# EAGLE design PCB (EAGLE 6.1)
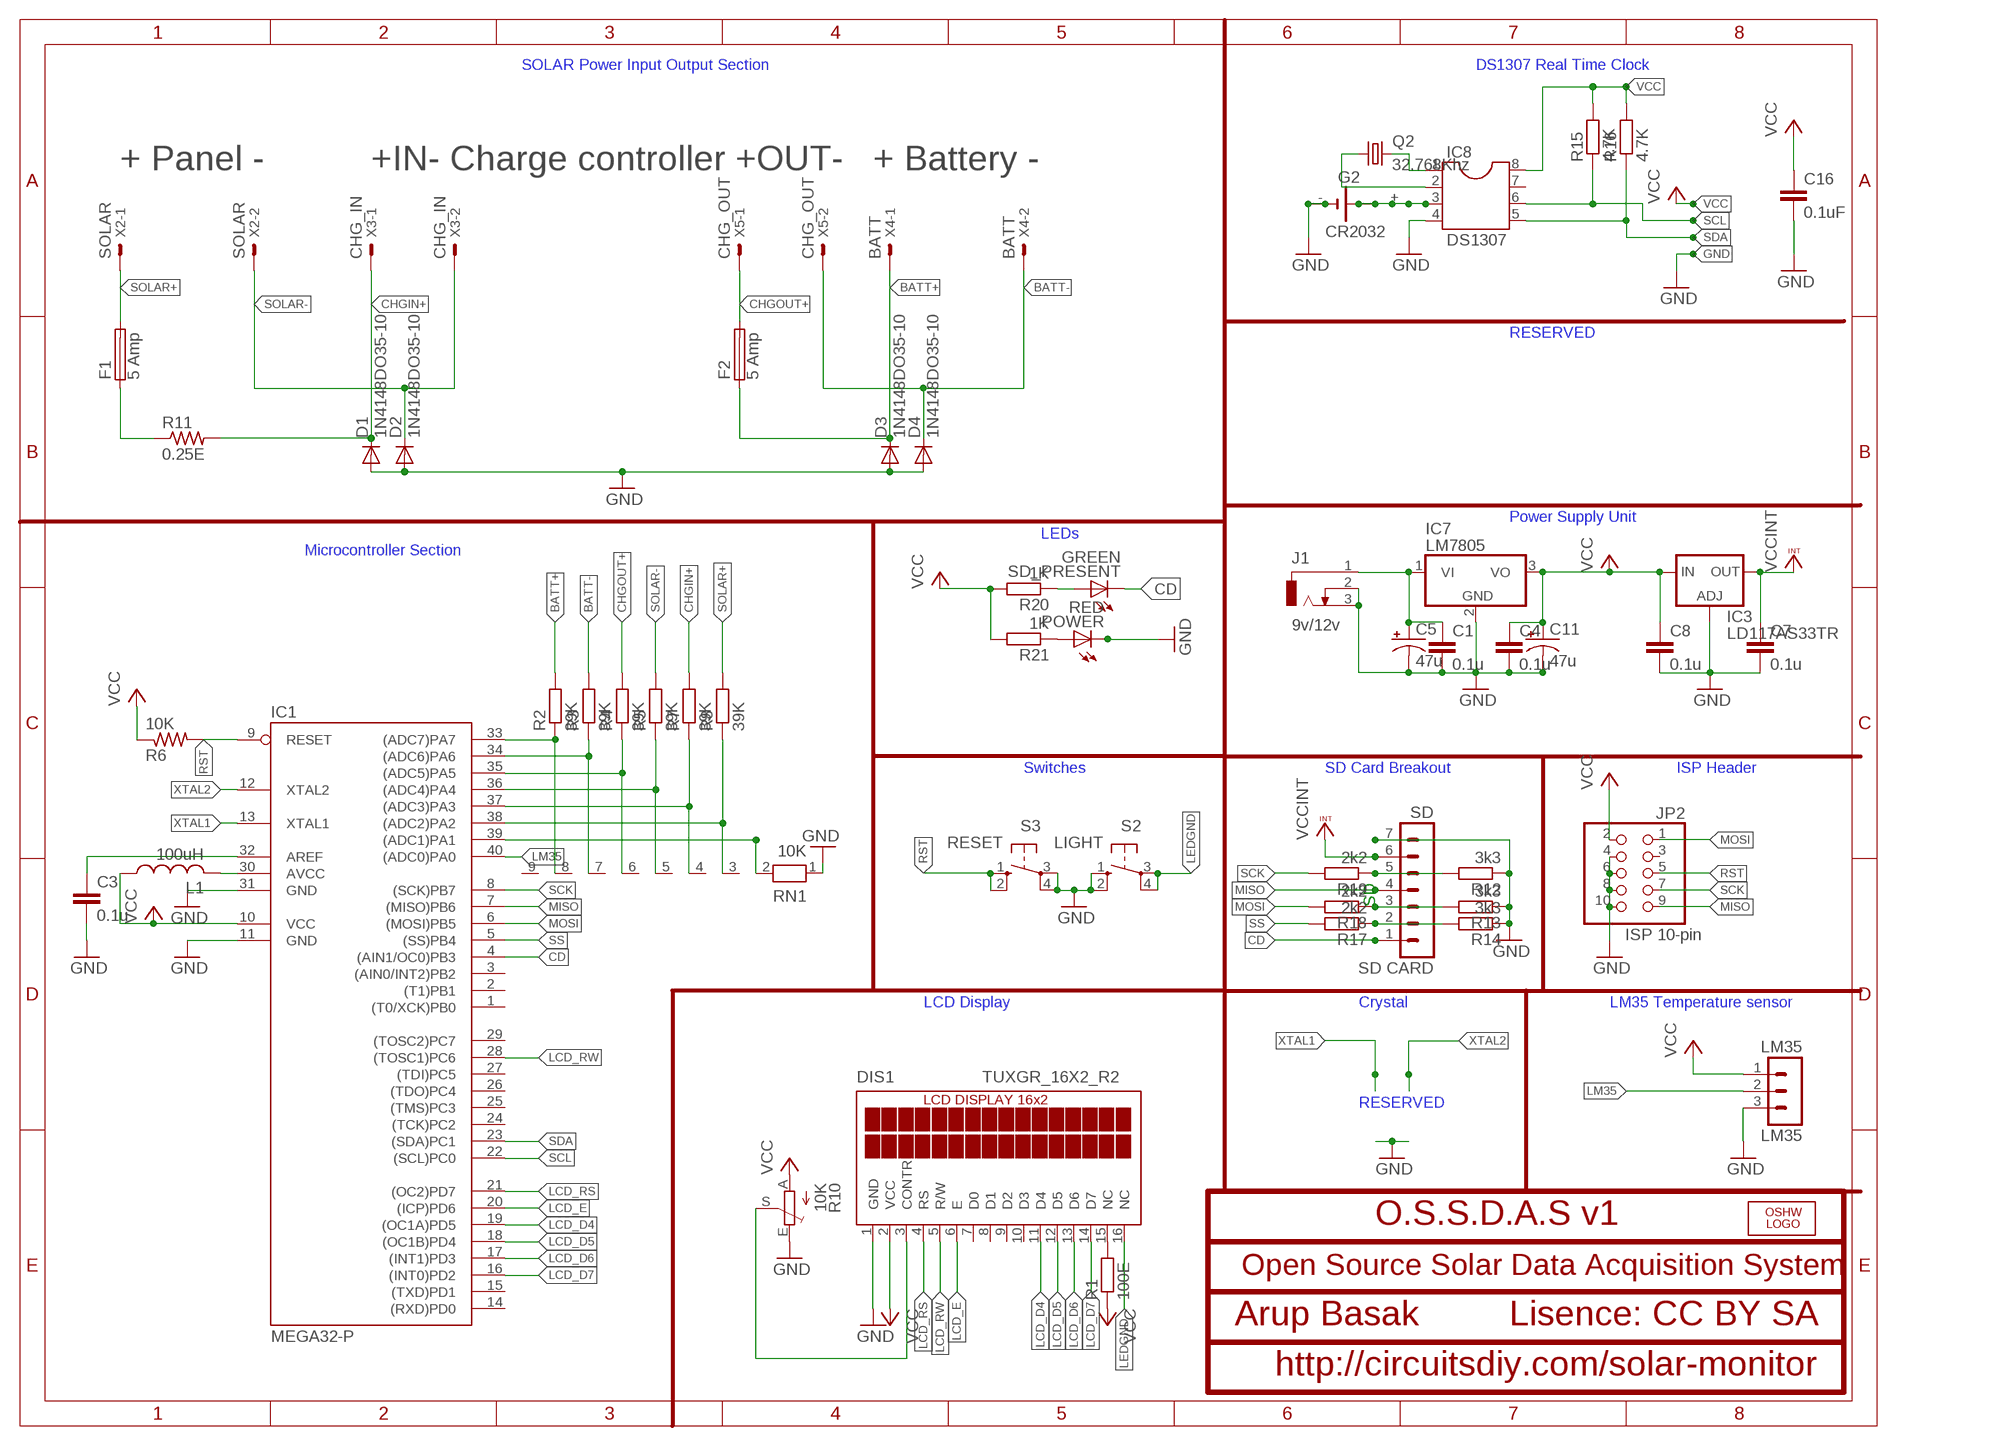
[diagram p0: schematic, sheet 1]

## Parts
C1  0.1u  C-EU025-025X050  [C025-025X050]
C3  0.1u  C-EU025-025X050  [C025-025X050]
C4  0.1u  C-EU025-025X050  [C025-025X050]
C5  47u  CPOL-USE2.5-7  [E2,5-7]
C7  0.1u  C-EU025-025X050  [C025-025X050]
C8  0.1u  C-EU025-025X050  [C025-025X050]
C11  47u  CPOL-USE2.5-7  [E2,5-7]
C16  0.1uF  C-EU050-024X044  [C050-024X044]
D1  1N4148DO35-10  [DO35-10]
D2  1N4148DO35-10  [DO35-10]
D3  1N4148DO35-10  [DO35-10]
D4  1N4148DO35-10  [DO35-10]
DIS1  TUXGR_16X2_R2  [TUXGR_16X2_R2]
F1  5 Amp  SH22,5A  [SH22,5A]
F2  5 Amp  SH22,5A  [SH22,5A]
G2  CR2032  B2430UNI  [B2430UNI]
IC1  MEGA32-P  [DIL40]
IC3  LD117AS33TR  [SOT223]
IC7  LM7805  7805TV  [TO220V]
IC8  DS1307  DIL8  [DIL08]
J1  9v/12v  DCJ0202  [DCJ0202]
JP2  ISP 10-pin  PINHD-2X5  [2X05]
L1  100uH  L-US0207/12  [0207/12]
LM35  LM35  MA03-1  [MA03-1]
LOGO1  OSHW_LOGO_FILLX0350-NT  [OSHW_FILLX350_NOTEXT]
POWER  RED  LED5MM  [LED5MM]
Q2  32.768Khz  CRYSTALTC38H  [TC38H]
R1  100E  R-EU_0207/7  [0207/7]
R2  39K  R-EU_0207/10  [0207/10]
R3  39K  R-EU_0207/10  [0207/10]
R4  39K  R-EU_0207/10  [0207/10]
R5  39K  R-EU_0207/10  [0207/10]
R6  10K  R-US_0207/10  [0207/10]
R7  39K  R-EU_0207/10  [0207/10]
R8  39K  R-EU_0207/10  [0207/10]
R10  10K  TRIM_EU-CA6V  [CA6V]
R11  0.25E  R-US_VTA53  [VTA53]
R12  3k3  R-EU_0207/10  [0207/10]
R13  3k3  R-EU_0207/10  [0207/10]
R14  3k3  R-EU_0207/10  [0207/10]
R15  4.7K  R-EU_0207/7  [0207/7]
R16  4.7K  R-EU_0207/7  [0207/7]
R17  2k2  R-EU_0207/10  [0207/10]
R18  2k2  R-EU_0207/10  [0207/10]
R19  2k2  R-EU_0207/10  [0207/10]
R20  1K  R-EU_0207/10  [0207/10]
R21  1K  R-EU_0207/10  [0207/10]
RN1  10K  RN08  [RN-9]
S2  LIGHT  10-XX  [B3F-10XX]
S3  RESET  10-XX  [B3F-10XX]
SD  SD CARD  MA07-1  [MA07-1]
SD_PRESENT  GREEN  LED5MM  [LED5MM]
X2  SOLAR  KK-156-2  [KK-156-2]
X3  CHG_IN  KK-156-2  [KK-156-2]
X4  BATT  KK-156-2  [KK-156-2]
X5  CHG_OUT  KK-156-2  [KK-156-2]

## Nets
AREF: C3.1 IC1.32(AREF)
AVCC: IC1.30(AVCC) L1.2
BATT+: D3.C F2.1 R2.2 X4.1
BATT-: D4.C R3.2 X4.2 X5.2
CD: IC1.4((AIN1/OC0)PB3) SD.1 SD_PRESENT.K(C)
CHGIN+: D1.C R7.2 R11.2 X3.1
CHGOUT+: F2.2 R4.2 X5.1
CS: R14.2 R17.1 SD.2
D1: R13.2 R18.1 SD.3
GND: C1.2 C3.2 C4.2 C5.- C7.2 C8.2 C11.- C16.2 D1.A D2.A D3.A D4.A DIS1.1(GND) G2.- G2.-@1(-) IC1.11(GND) IC1.31(GND) IC3.1(ADJ) IC7.2(GND) IC8.4 J1.2 J1.3 JP2.4 JP2.6 JP2.8 JP2.10 LM35.3 POWER.K(C) R10.E R12.1 R13.1 R14.1 RN1.1 S2.1(S) S2.2(S1) S3.3(P) S3.4(P1) SD.7
LCD_D4: DIS1.11(D4) IC1.19((OC1A)PD5)
LCD_D5: DIS1.12(D5) IC1.18((OC1B)PD4)
LCD_D6: DIS1.13(D6) IC1.17((INT1)PD3)
LCD_D7: DIS1.14(D7) IC1.16((INT0)PD2)
LCD_E: DIS1.6(E) IC1.20((ICP)PD6)
LCD_RS: DIS1.4(RS) IC1.21((OC2)PD7)
LCD_RW: DIS1.5(R/W) IC1.28((TOSC1)PC6)
LEDGND: DIS1.16(NC) S2.3(P) S2.4(P1)
LM35: IC1.40((ADC0)PA0) LM35.2
MISO: IC1.7((MISO)PB6) JP2.9 SD.4
MOSI: IC1.6((MOSI)PB5) JP2.1 R18.2
N$2: DIS1.15(NC) R1.2
N$3: IC1.33((ADC7)PA7) R2.1 RN1.8
N$4: DIS1.3(CONTR) R10.S
N$5: IC1.34((ADC6)PA6) R3.1 RN1.7
N$6: IC1.35((ADC5)PA5) R4.1 RN1.6
N$7: IC1.36((ADC4)PA4) R5.1 RN1.5
N$8: IC8.1 Q2.2
N$9: IC1.37((ADC3)PA3) R7.1 RN1.4
N$10: IC1.38((ADC2)PA2) R8.1 RN1.3
N$11: IC1.39((ADC1)PA1) RN1.2
N$12: IC8.2 Q2.1
N$16: G2.+ G2.+@1(+) G2.+@2(+) G2.+@3(+) G2.+@4(+) IC8.3
N$17: F1.1 R11.1
N$22: R20.1 SD_PRESENT.A
N$23: POWER.A R21.1
N$24: C1.1 C5.+ IC7.1(VI) J1.1
RST: IC1.9(RESET) JP2.5 R6.2 S3.1(S) S3.2(S1)
SCK: IC1.8((SCK)PB7) JP2.7 R19.2
SCL: IC1.22((SCL)PC0) IC8.6 R15.1
SD_SCK: R12.2 R19.1 SD.5
SDA: IC1.23((SDA)PC1) IC8.5 R16.1
SOLAR+: F1.2 R8.2 X2.1
SOLAR-: D2.C R5.2 X2.2 X3.2
SS: IC1.5((SS)PB4) R17.2
VCC: C4.1 C8.1 C11.+ C16.1 DIS1.2(VCC) IC1.10(VCC) IC3.3(IN) IC7.3(VO) IC8.8 JP2.2 L1.1 LM35.1 R1.1 R6.1 R10.A R15.2 R16.2 R20.2 R21.2
VCCINT: C7.1 IC3.4(OUT) SD.6
XTAL1: IC1.13(XTAL1)
XTAL2: IC1.12(XTAL2)
Unconnected: DIS1.7(D0) DIS1.8(D1) DIS1.9(D2) DIS1.10(D3) IC1.1((T0/XCK)PB0) IC1.2((T1)PB1) IC1.3((AIN0/INT2)PB2) IC1.14((RXD)PD0) IC1.15((TXD)PD1) IC1.24((TCK)PC2) IC1.25((TMS)PC3) IC1.26((TDO)PC4) IC1.27((TDI)PC5) IC1.29((TOSC2)PC7) IC8.7 JP2.3 RN1.9

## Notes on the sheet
- SOLAR Power Input Output Section | DS1307 Real Time Clock
- + Panel - | +IN- Charge controller +OUT- | + Battery -
- RESERVED
- Power Supply Unit
- LEDs
- Microcontroller Section
- Switches | SD Card Breakout | ISP Header
- SD
- LCD Display | Crystal | LM35 Temperature sensor
- RESERVED
- O.S.S.D.A.S v1
- Open Source Solar Data Acquisition System
- Arup Basak | Lisence: CC BY SA
- http://circuitsdiy.com/solar-monitor

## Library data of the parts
C1 C3 C4 C7 C8 = resistor:C-EU: CAPACITOR, European symbol
C5 C11 = resistor:CPOL-US: POLARIZED CAPACITOR, American symbol
C16 = rcl:C-EU: CAPACITOR, European symbol
D1-D4 = diode:1N4148: DIODE
DIS1 = display-lcd:TUXGR_16X2_R2: Tuxgraphics LCD display 16x2 characters reflective, without background light Source: tuxgr_12x2_r2.pdf; OC_FARNELL: unknown; OC_NEWARK: unknown
F1 F2 = fuse:SH22,5A: FUSE HOLDER; MPN: 0031.7701.11; OC_FARNELL: unknown; OC_NEWARK: 04F1224
G2 = battery:B2430UNI: LI BATTERY
IC1 = atmel:MEGA32-P: MICROCONTROLLER 32 Kbytes FLASH 2 Kbytes SRAM 1 Kbytes EEPROM USART 8-channel 10 bit ADC Source: www.atmel.com .. doc2503.pdf
IC3 = v-reg:LD117A?*: Low drop fixed and adjustable positive voltage regulators 1 A Source: http://www.st.com/stonline/products/literature/ds/7194/ld1117axx.pdf
IC7 = linear:78*: Positive VOLTAGE REGULATOR Source: http://cache.national.com/ds/LM/LM78L05.pdf http://www.fairchildsemi.com/ds/LM/LM7805.pdf
IC8 = ic-package:DIL8: Dual In Line / Socket
J1 = con-jack:DCJ0202: DC POWER JACK Source: DCJ0202.pdf
JP2 = sonar:PINHD-2X5: PIN HEADER
L1 = resistor:L-US: INDUCTOR, American symbol
LM35 = con-lstb:MA03-1: PIN HEADER
LOGO1 = ohw-logo:OSHW_LOGO_FILL
POWER SD_PRESENT = led:LED: LED
Q2 = crystal:CRYSTAL: CRYSTAL
R1-R5 R7 R8 R15 R16 R20 R21 = rcl:R-EU_: RESISTOR, European symbol
R6 = resistor:R-US_: RESISTOR, American symbol
R10 = pot:TRIM_EU-: POTENTIOMETER
R11 = rcl:R-US_: RESISTOR, American symbol
R12-R14 R17-R19 = resistor:R-EU_: RESISTOR, European symbol
RN1 = resistor-net:RN08: RESISTOR NETWORK
S2 S3 = switch-omron:10-XX: OMRON SWITCH
SD = con-lstb:MA07-1: PIN HEADER
X2-X5 = con-molex:KK-156-2: KK 156 HEADER; OC_FARNELL: unknown; OC_NEWARK: unknown

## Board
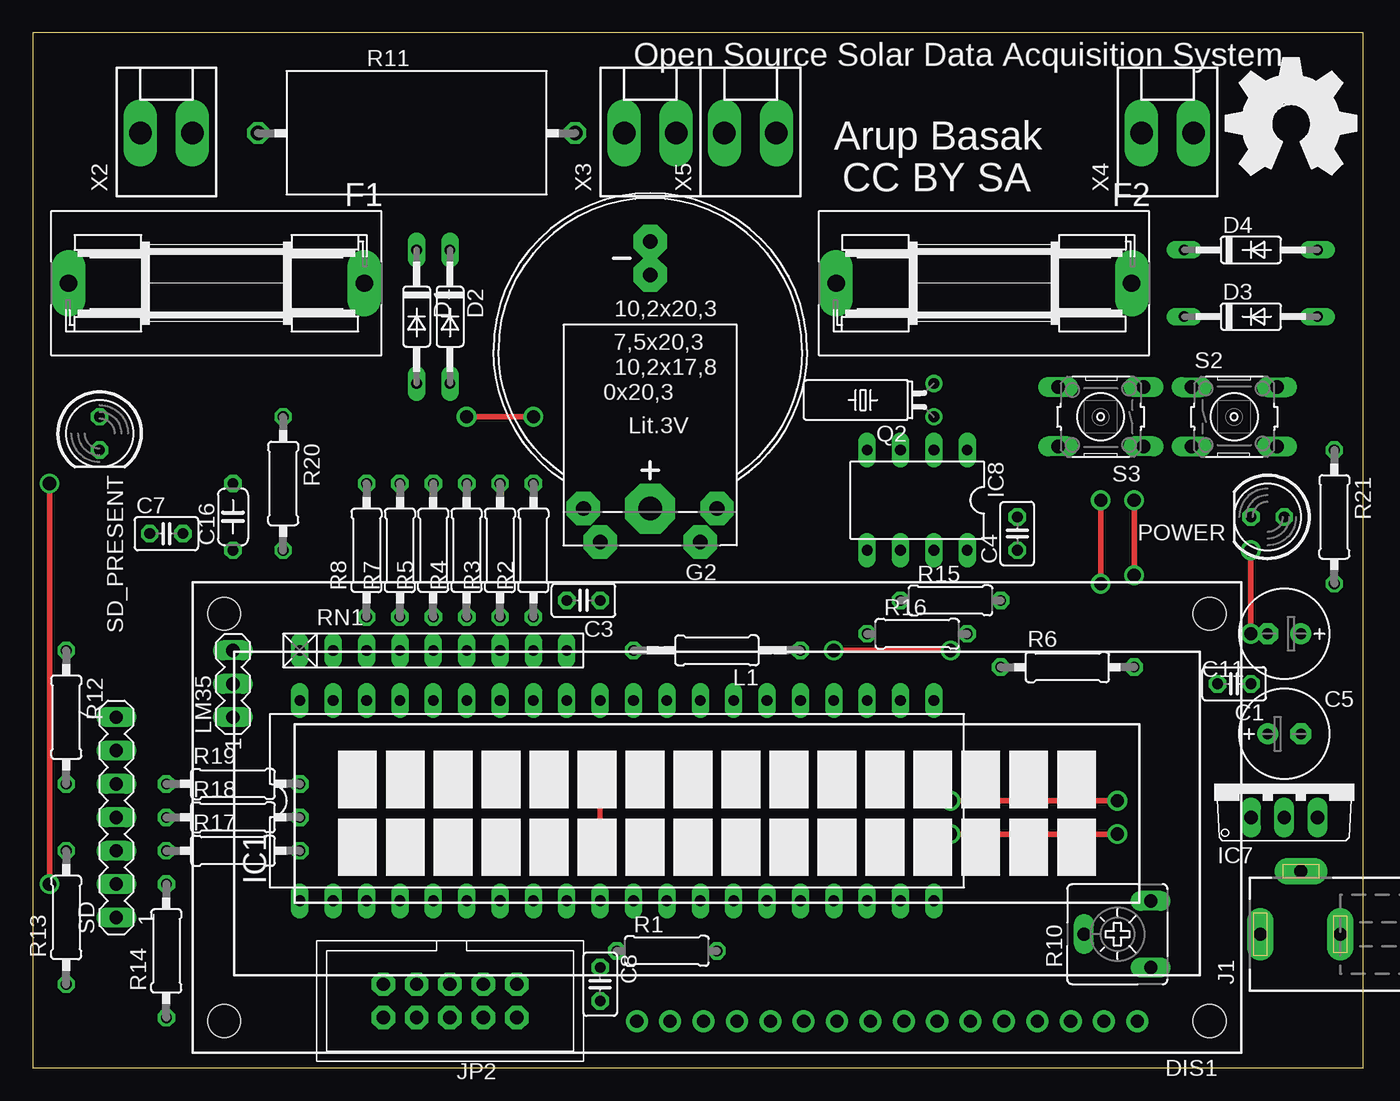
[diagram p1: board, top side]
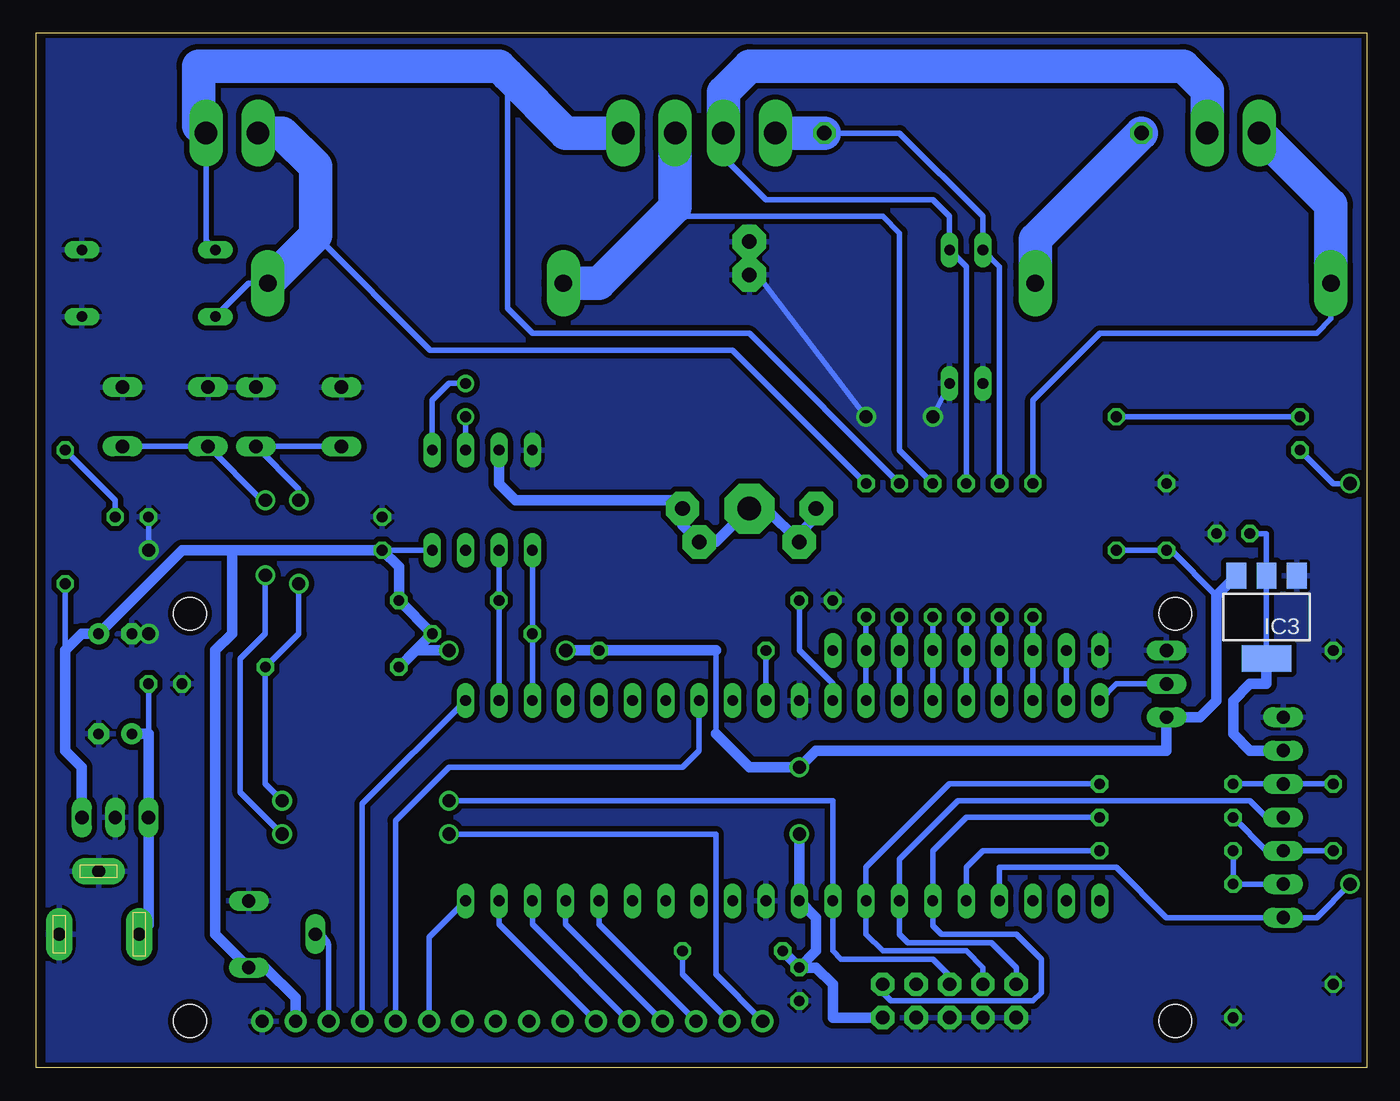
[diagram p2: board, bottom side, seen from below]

Size 101.27 x 78.73 mm. Coordinates in mm from the lower left corner, seen from the top.
Outline: 0,0 101.27,0 101.27,78.73 0,78.73 0,0
Copper layers (1*16): Top 0.035mm / dielectric 1.5mm / Bottom 0.035mm
Design rules: minimum track width 6mil, minimum drill 12mil, track to track 6mil, track to pad 6mil, pad to pad 6mil, via to via 6mil, smd to smd 0mil, copper to edge 10mil, drill to drill 10mil, minimum pad ring 10mil, minimum via ring 6mil, stop-mask expansion 2mil, vias tented up to drill 100mil, thermal gap 10mil

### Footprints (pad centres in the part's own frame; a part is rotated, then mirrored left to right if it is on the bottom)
C025-025X050 = drill 0.813 octagon: 1 -1.27,0; 2 1.27,0
E2,5-7 = drill 0.813 pad 1.6: + -1.27,0 | drill 0.813 pad 1.6 octagon: - 1.27,0
C050-024X044 = drill 0.813 octagon: 1 -2.54,0; 2 2.54,0
DO35-10 = drill 0.813 long: A 5.08,0; C -5.08,0
TUXGR_16X2_R2 = drill 1 pad 1.676: 1 -32,15.5; 2 -29.46,15.5; 3 -26.92,15.5; 4 -24.38,15.5; 5 -21.84,15.5; 6 -19.3,15.5; 7 -16.76,15.5; 8 -14.22,15.5; 9 -11.68,15.5; 10 -9.14,15.5; 11 -6.6,15.5; 12 -4.06,15.5; 13 -1.52,15.5; 14 1.02,15.5; 15 3.56,15.5; 16 6.1,15.5 | hole 2.5: -37.5,-15.5; 37.5,-15.5; -37.5,15.5; 37.5,15.5
SH22,5A = drill 1.321 pad 2.54 long: 1 -11.252,0; 2 11.252,0
B2430UNI = drill 1.118 pad 2.54 octagon: + 3.81,14.605; +@1 -3.81,14.605; +@2 -5.08,12.065; +@3 5.08,12.065; - 0,-5.715; -@1 0,-8.255 | drill 1.803 pad 3.81 octagon: +@4 0,12.065
DIL40 = drill 0.813 long: 1 -24.13,-7.62; 2 -21.59,-7.62; 3 -19.05,-7.62; 4 -16.51,-7.62; 5 -13.97,-7.62; 6 -11.43,-7.62; 7 -8.89,-7.62; 8 -6.35,-7.62; 9 -3.81,-7.62; 10 -1.27,-7.62; 11 1.27,-7.62; 12 3.81,-7.62; 13 6.35,-7.62; 14 8.89,-7.62; 15 11.43,-7.62; 16 13.97,-7.62; 17 16.51,-7.62; 18 19.05,-7.62; 19 21.59,-7.62; 20 24.13,-7.62; 21 24.13,7.62; 22 21.59,7.62; 23 19.05,7.62; 24 16.51,7.62; 25 13.97,7.62; 26 11.43,7.62; 27 8.89,7.62; 28 6.35,7.62; 29 3.81,7.62; 30 1.27,7.62; 31 -1.27,7.62; 32 -3.81,7.62; 33 -6.35,7.62; 34 -8.89,7.62; 35 -11.43,7.62; 36 -13.97,7.62; 37 -16.51,7.62; 38 -19.05,7.62; 39 -21.59,7.62; 40 -24.13,7.62
SOT223 = smd 1.5 x 2: 1 -2.3,-3.15; 2 0,-3.15; 3 2.3,-3.15 | smd 3.8 x 2: 4 0,3.15
TO220V = drill 1.016 long: 1 -2.54,-2.54; 2 0,-2.54; 3 2.54,-2.54
DIL08 = drill 0.813 long: 1 -3.81,-3.81; 2 -1.27,-3.81; 3 1.27,-3.81; 4 3.81,-3.81; 5 3.81,3.81; 6 1.27,3.81; 7 -1.27,3.81; 8 -3.81,3.81
DCJ0202 = drill 1 pad 2 long: 1 0,3.1; 2 4.8,0; 3 0,-3
2X05 = drill 1.016 pad 1.778 octagon: 1 -5.08,-1.27; 2 -5.08,1.27; 3 -2.54,-1.27; 4 -2.54,1.27; 5 0,-1.27; 6 0,1.27; 7 2.54,-1.27; 8 2.54,1.27; 9 5.08,-1.27; 10 5.08,1.27
0207/12 = drill 0.813 octagon: 1 -6.35,0; 2 6.35,0
MA03-1 = drill 1.016 long: 1 -2.54,0; 2 0,0; 3 2.54,0
LED5MM = drill 0.813 octagon: A -1.27,0; K 1.27,0
TC38H = drill 0.813: 1 -1.27,0; 2 1.27,0
0207/7 = drill 0.813 octagon: 1 -3.81,0; 2 3.81,0
0207/10 = drill 0.813 octagon: 1 -5.08,0; 2 5.08,0
CA6V = drill 1.016 long: A -2.54,-2.54; E 2.54,-2.54; S 0,2.54
VTA53 = drill 1.1 octagon: 1 -12.065,0; 2 12.065,0
RN-9 = drill 0.813 long: 1 -10.16,0; 2 -7.62,0; 3 -5.08,0; 4 -2.54,0; 5 0,0; 6 2.54,0; 7 5.08,0; 8 7.62,0; 9 10.16,0
B3F-10XX = drill 1.016 long: 1 -3.251,2.261; 2 3.251,2.261; 3 -3.251,-2.261; 4 3.251,-2.261
MA07-1 = drill 1.016 long: 1 -7.62,0; 2 -5.08,0; 3 -2.54,0; 4 0,0; 5 2.54,0; 6 5.08,0; 7 7.62,0
KK-156-2 = drill 1.7 pad 2.184 long: 1 -1.98,0; 2 1.98,0

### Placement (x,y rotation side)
C1  91.44,29.21 180 top
C3  41.91,35.56 180 top
C4  74.93,40.64 90 top
C5  95.25,25.4 0 top
C7  10.16,40.64 0 top
C8  43.18,6.35 270 top
C11  95.25,33.02 180 top
C16  15.24,41.91 90 top
D1  29.21,57.15 270 top
D2  31.75,57.15 270 top
D3  92.71,57.15 0 top
D4  92.71,62.23 0 top
DIS1  52.07,19.05 180 top
F1  13.97,59.69 180 top
F2  72.39,59.69 180 top
G2  46.99,54.61 180 top
IC1  44.45,20.32 0 top
IC3  7.62,34.29 180 bottom
IC7  95.25,21.59 0 top
IC8  67.31,43.18 180 top
J1  96.52,10.16 90 top
JP2  31.75,5.08 180 top
L1  52.07,31.75 180 top
LM35  15.24,29.21 90 top
LOGO1  90.81,67.95 0 top
POWER  93.98,41.91 180 top
Q2  68.58,50.8 90 top
R1  48.26,8.89 0 top
R2  38.1,39.37 90 top
R3  35.56,39.37 90 top
R4  33.02,39.37 90 top
R5  30.48,39.37 90 top
R6  78.74,30.48 0 top
R7  27.94,39.37 90 top
R8  25.4,39.37 90 top
R10  82.55,10.16 90 top
R11  29.21,71.12 0 top
R12  2.54,26.67 270 top
R13  2.54,11.43 90 top
R14  10.16,8.89 90 top
R15  69.85,35.56 0 top
R16  67.31,33.02 0 top
R17  15.24,16.51 0 top
R18  15.24,19.05 0 top
R19  15.24,21.59 0 top
R20  19.05,44.45 270 top
R21  99.06,41.91 270 top
RN1  30.48,31.75 0 top
S2  91.44,49.53 0 top
S3  81.28,49.53 180 top
SD  6.35,19.05 90 top
SD_PRESENT  5.08,48.26 270 top
X2  10.16,71.12 0 top
X3  46.99,71.12 0 top
X4  86.36,71.12 0 top
X5  54.61,71.12 0 top

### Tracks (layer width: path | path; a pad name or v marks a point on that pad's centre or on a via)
AREF
  Bottom 0.406: IC1.32 40.64,29.21 43.18,31.75 C3.1
AVCC
  Bottom 0.406: L1.2 IC1.30
BATT+
  Bottom 0.406: 80.01,63.32 71.3,54.61 48.26,54.61 R2.2 | 83.64,60.78 F2.1 85.09,59.69 D3.C
  Bottom 2.54: F2.1 80.01,63.32 80.01,68.58 82.55,71.12 X4.1
BATT-
  Bottom 0.406: R3.2 46.99,55.88 63.5,55.88 65.41,57.78 65.41,75.56 | D4.C 88.34,62.94 X4.2
  Bottom 2.54: X5.2 60.96,71.12 65.41,75.56 66.04,76.2 88.9,76.2 88.9,71.68 X4.2
CD  (via drill 1 pad 1.27)
  Top 0.406: v1.27,44.45 v1.27,13.97
  Bottom 0.406: IC1.4 27.94,15.24 19.05,15.24 15.24,11.43 SD.1 3.81,11.43 v1.27,13.97 | SD_PRESENT.K 2.54,44.45 v1.27,44.45
CHGIN+
  Bottom 0.406: R11.2 35.56,71.12 29.21,64.77 D1.C 27.94,60.96 R7.2
  Bottom 2.54: R11.2 X3.1
CHGOUT+
  Bottom 0.406: R4.2 35.56,46.99 35.56,63.5 36.83,64.77 52.07,64.77 52.63,65.33 52.63,65.48
  Bottom 2.54: X5.1 52.63,65.48 58.42,59.69 F2.2
CS
  Bottom 0.406: SD.2 R14.2 R17.1
D1
  Bottom 0.406: R13.2 SD.3 7.62,16.51 R18.1
GND  (via drill 1 pad 1.27)
  Top 0.406: v33.02,49.53 v38.1,49.53 | v92.71,33.02 v92.71,39.37
  Bottom 0.406: D2.A v33.02,49.53 | v38.1,49.53 46.35,60.32 G2.- | C11.- v92.71,33.02 | v92.71,39.37 POWER.K
  pour Bottom (isolate 0.406): 0,78.74 100.33,78.74 100.33,0 0,0
LCD_D4
  Bottom 0.406: IC1.19 66.04,10.92 DIS1.11
LCD_D5
  Bottom 0.406: IC1.18 63.5,10.92 DIS1.12
LCD_D6
  Bottom 0.406: IC1.17 60.96,10.92 DIS1.13
LCD_D7
  Bottom 0.406: IC1.16 58.42,10.92 DIS1.14
LCD_E
  Bottom 0.406: IC1.20 71.37,9.91 DIS1.6
LCD_RS
  Bottom 0.406: IC1.21 76.45,20.07 DIS1.4
LCD_RW
  Bottom 0.406: IC1.28 50.8,24.13 52.07,22.86 69.85,22.86 73.91,18.8 DIS1.5
LEDGND  (via drill 1 pad 1.27)
  Top 0.406: v69.85,17.78 v82.55,17.78 | v83.82,37.46 v83.82,43.18
  Bottom 0.406: DIS1.16 49.53,7.11 49.53,17.78 v69.85,17.78 | v82.55,17.78 85.72,20.96 85.72,31.11 83.82,33.02 v83.82,37.46 | S2.4 S2.3 84.1,43.18 v83.82,43.18
LM35
  Bottom 0.406: IC1.40 19.05,29.21 LM35.2
MISO
  Bottom 0.406: SD.4 7.62,19.05 8.89,20.32 31.11,20.32 35.56,15.88 IC1.7 35.56,10.16 34.92,9.53 28.57,9.53 26.67,7.62 JP2.9
MOSI
  Bottom 0.406: R18.2 30.48,19.05 33.02,16.51 IC1.6 33.02,10.79 32.38,10.16 26.67,10.16 24.77,8.26 24.77,5.71 25.4,5.08 36.2,5.08 36.83,5.71 JP2.1
N$2
  Bottom 0.406: DIS1.15 52.07,7.11 R1.2
N$3
  Bottom 0.406: IC1.33 RN1.8 R2.1
N$4
  Bottom 0.406: DIS1.3 78.99,9.14 arc-90 R10.S
N$5
  Bottom 0.406: IC1.34 RN1.7 R3.1
N$6
  Bottom 0.406: IC1.35 RN1.6 R4.1
N$7
  Bottom 0.406: IC1.36 RN1.5 R5.1
N$8
  Bottom 0.406: IC8.1 71.12,50.8 69.85,52.07 Q2.2
N$9
  Bottom 0.406: IC1.37 RN1.4 R7.1
N$10
  Bottom 0.406: IC1.38 RN1.3 R8.1
N$11
  Bottom 0.406: IC1.39 RN1.2
N$12
  Bottom 0.406: Q2.1 IC8.2
N$16
  Bottom 0.813: IC8.3 66.04,44.45 64.77,43.18 52.7,43.18 G2.+@2 52.07,41.27 G2.+@1 49.53,40 G2.+@4 45.72,42.54 G2.+ 43.18,40.64 41.91,41.91 G2.+@3
N$17
  Bottom 2.54: R11.1 25.22,63.04 F1.1
N$22
  Bottom 0.406: R20.1 SD_PRESENT.A
N$23
  Bottom 0.406: R21.1 95.25,43.18 POWER.A
N$24
  Bottom 0.406: 92.71,25.4 C1.1
  Bottom 0.813: J1.1 92.71,10.87 IC7.1 92.71,25.4 C5.+
RST  (via drill 1 pad 1.27)
  Top 0.406: v69.85,20.32 v82.55,20.32 | v81.28,36.83 v81.28,43.18
  Bottom 0.406: JP2.5 31.75,6.99 33.02,8.26 40.01,8.26 40.64,8.89 IC1.9 40.64,20.32 v69.85,20.32 | v82.55,20.32 83.82,21.59 R6.2 81.28,33.02 v81.28,36.83 | S3.2 S3.1 81.28,44.02 v81.28,43.18
SCK
  Bottom 0.406: R19.2 31.75,21.59 38.1,15.24 IC1.8 38.1,10.16 36.83,8.89 30.48,8.89 29.21,7.62 JP2.7
SCL
  Bottom 0.406: IC1.22 R15.1 IC8.6
SD_SCK
  Bottom 0.406: R12.2 SD.5 R19.1
SDA
  Bottom 0.406: IC1.23 R16.1 IC8.5
SOLAR+
  Bottom 0.406: R8.2 25.4,50.8 20.32,55.88 3.81,55.88 2.72,56.97 F1.2
  Bottom 2.54: F1.2 2.72,65.66 X2.1
SOLAR-
  Bottom 0.406: X3.2 48.97,69.29 45.72,66.04 33.02,66.04 31.75,64.77 D2.C 30.48,60.96 R5.2
  Bottom 2.54: X3.2 48.97,74.22 46.99,76.2 13.97,76.2 12.14,74.37 X2.2
SS
  Bottom 0.406: R17.2 29.21,16.51 30.48,15.24 IC1.5
VCC  (via drill 1 pad 1.27)
  Top 0.406: v60.96,31.75 v69.85,31.75 | v43.18,22.86 v43.18,17.78
  Bottom 0.406: IC8.8 C4.1 | R21.2 99.06,31.75 | 49.53,31.75 49.53,25.4 | 11.43,35.93 14.87,39.37 C16.1 R20.2
  Bottom 0.813: C8.1 41.91,8.89 41.91,11.43 IC1.10 v43.18,17.78 | DIS1.2 81.53,5.33 83.82,7.62 R10.A 87.63,10.16 87.63,31.75 86.36,33.02 86.36,39.37 | IC7.3 97.79,22.86 99.06,24.13 99.06,31.75 97.79,33.02 C11.+ 90.17,39.37 86.36,39.37 | 86.36,39.37 C4.1 73.66,38.1 R15.2 R16.2 R6.1 72.39,31.75 v69.85,31.75 | v60.96,31.75 L1.1 49.53,31.75 | R1.1 C8.1 | JP2.2 40.64,3.81 40.64,6.35 41.91,7.62 C8.1 | 49.53,25.4 46.99,22.86 v43.18,22.86 41.91,24.13 15.24,24.13 LM35.1 12.7,26.67 11.43,27.94 11.43,35.93 IC3.3
VCCINT
  Bottom 0.406: IC3.4 7.64,40.64 C7.1
  Bottom 0.813: SD.6 8.89,24.13 10.16,25.4 10.16,27.94 8.89,29.21 7.62,29.21 IC3.4

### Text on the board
tPlace: Open Source Solar Data Acquisition System | Arup Basak | CC BY SA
